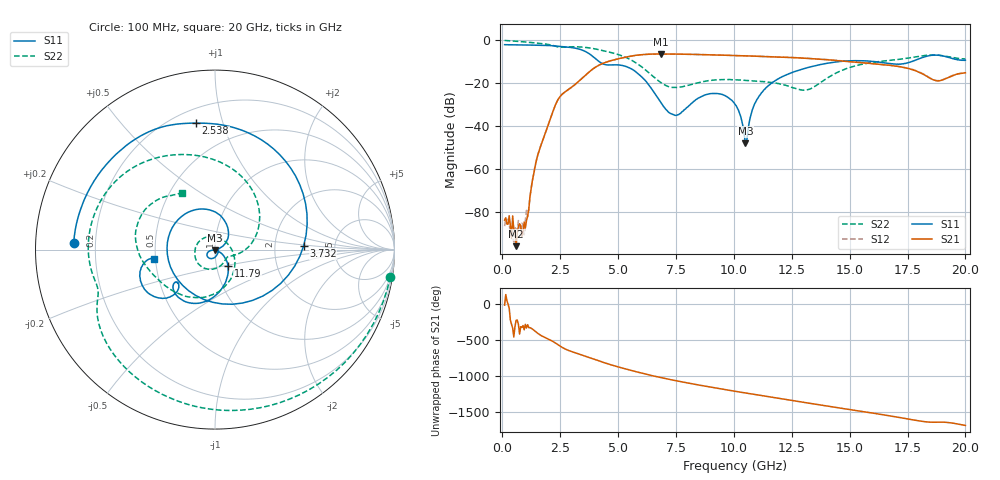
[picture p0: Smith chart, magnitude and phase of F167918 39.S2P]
!  2-Port S-parameters saved by WinCal
! VAR MeasName=S-Parameters (CALIBRATED_DATA) read from VNA (N5242A)
! VAR MeasDate=2016-11-22 10:26:37
! VAR NAME=F167918 39
! VAR FILENAME=F167918 39.S2P
! VAR DATE=2016-11-22 10:26:37
! VAR PHYS_PORTS=1,2
# Hz S DB R 50
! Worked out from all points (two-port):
!   401 points, 100 MHz to 20 GHz, reference 50 ohm
!   highest |S21| = -6.38 dB at 6.866 GHz (marker M1); lowest = -95.7 dB at 597.5 MHz (marker M2)
!   |S21| within 3 dB of the highest: 4.734 GHz to 14.38 GHz (9.641 GHz wide, 101 % of centre)
!   lowest |S11| = -47.8 dB at 10.5 GHz (marker M3), VSWR 1.01, Z = 49.8 - j0.329 ohm
!   |S11| at or under -10 dB: 4.191 GHz to 14.49 GHz (10.3 GHz wide, 110 % of centre); 16.14 GHz to 17.66 GHz (1.515 GHz wide, 8.97 % of centre)
!   |S22| runs from -23.2 to -0.1 dB; largest |S21 - S12| = 0.0044
!   S11 on the Smith chart (normalised r, x): 100 MHz: 0.12, +0.02; 2.538 GHz: 0.29, +0.82; 3.732 GHz: 2.95, +0.17; 11.79 GHz: 1.14, -0.21; 20 GHz: 0.49, -0.06
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1e8  -2.07 177.3  -83.62 -19.9  -86.44 100.3  -0.10 -8.8
5.975e8  -2.13 164.0  -95.75 130.5  -87.64 117.1  -0.45 -48.6
1.04525e9  -2.21 151.8  -83.84 24.3  -79.11 -7.1  -0.86 -81.1
1.5925e9  -2.33 135.4  -51.26 -62.5  -51.18 -63.2  -1.43 -116.1
2.53775e9  -2.94 98.5  -25.63 125.0  -25.63 124.7  -3.25 -162.4
3.43325e9  -4.51 37.4  -17.78 11.6  -17.80 11.7  -3.17 158.1
3.73175e9  -6.12 2.5  -14.88 -20.5  -14.88 -20.3  -3.51 143.2
4.1795e9  -9.91 -72.4  -11.56 -71.4  -11.51 -71.3  -4.42 121.1
4.677e9  -11.49 -166.7  -9.55 -123.7  -9.50 -124.0  -5.67 96.8
5.62225e9  -13.58 89.4  -7.26 152.4  -7.27 152.1  -9.53 42.7
6.7665e9  -27.60 22.5  -6.38 63.5  -6.40 63.5  -19.05 -16.5
6.866e9  -29.26 20.3  -6.38 56.7  -6.41 56.6  -19.79 -19.6
8.06e9  -30.44 -66.8  -6.54 -19.8  -6.55 -19.8  -20.89 -63.2
9.10475e9  -24.74 -127.4  -6.83 -80.0  -6.81 -80.2  -18.54 -115.8
1.005e10  -29.76 -164.9  -7.11 -131.5  -7.12 -131.4  -18.42 -151.2
1.049775e10  -47.84 -125.4  -7.25 -154.9  -7.26 -155.0  -18.71 -163.5
1.099525e10  -27.55 -30.6  -7.42 179.2  -7.41 179.2  -19.07 -176.6
1.179125e10  -18.73 -51.4  -7.71 138.0  -7.70 138.2  -19.90 157.0
1.338325e10  -12.18 -86.6  -8.57 56.7  -8.49 56.9  -22.16 23.9
1.67165e10  -10.83 -140.7  -11.60 -110.7  -11.63 -110.9  -9.37 -142.5
1.875625e10  -6.93 -155.6  -18.86 160.6  -18.72 160.0  -6.88 154.1
2e10  -9.29 -170.8  -15.14 115.5  -15.07 114.8  -8.69 120.4
